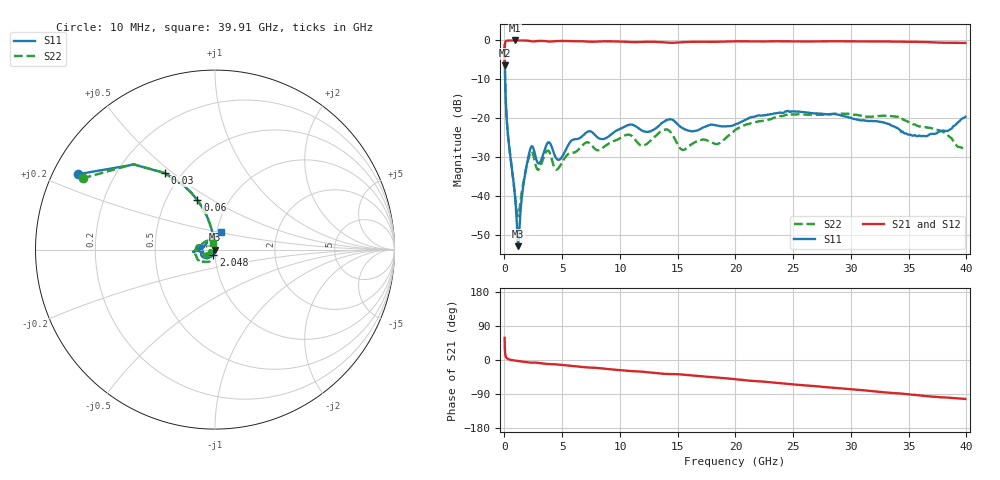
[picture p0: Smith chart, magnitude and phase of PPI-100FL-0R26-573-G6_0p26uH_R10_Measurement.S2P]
! Data measured by Modelithics Inc.  support@modelithics.com  813-866-6335  Tampa FL USA June 2025
! PPI-100FL-0R26-573-G6_0p26uH measured on 10-mil thick RO4350B board, mounted in 2-port shunt configuration on a 50-ohm transmission line
# Hz S MA R 50
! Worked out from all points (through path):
!   429 points, 10 MHz to 39.91 GHz, reference 50 ohm
!   highest |S21| = -0.03 dB at 882.5 MHz (marker M1); lowest = -6.4 dB at 10 MHz (marker M2)
!   group delay of S21, straight-line fit = 7.42 ps
!   lowest |S11| = -53.0 dB at 1.174 GHz (marker M3), VSWR 1.00, Z = 49.8 + j0.049 ohm
!   |S11| at or under -10 dB: 55.02 MHz to end of sweep
!   |S22| runs from -45.3 to -1.5 dB; largest |S21 - S12| = 0.024
!   S11 on the Smith chart (normalised r, x): 10 MHz: 0.07, +0.26; 30 MHz: 0.41, +0.47; 60 MHz: 0.71, +0.43; 2.048 GHz: 0.98, -0.06; 39.91 GHz: 1.05, +0.21
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1e7  0.8714 151.2  0.4784 58.5  0.4784 58.5  0.8372 151.7
3e7  0.5098 123.3  0.836 30.6  0.8361 30.6  0.5119 123.4
6e7  0.2921 109.5  0.9426 16.8  0.9427 16.8  0.2927 109.7
2e8  0.09232 98.5  0.9899 4.8  0.9899 4.8  0.09258 98.7
8.825328e8  0.01074 104.1  0.9961 -1.5  0.9962 -1.4  0.01119 113.4
1.173799e9  0.002238 167.3  0.9961 -2.7  0.9963 -2.7  0.005436 173.8
2.047598e9  0.0307 -106.3  0.9881 -6.3  0.9883 -6.3  0.0287 -132.0
2.435953e9  0.04288 -139.2  0.9679 -7.0  0.9681 -7.0  0.03559 -162.9
2.921397e9  0.02605 -141.1  0.9812 -7.7  0.9814 -7.7  0.02148 -155.4
3.795197e9  0.04875 -136.9  0.966 -10.6  0.966 -10.6  0.03811 -159.4
4.571907e9  0.02922 -143.5  0.9789 -11.8  0.9791 -11.8  0.02177 -149.8
6.70786e9  0.05777 -128.0  0.9723 -18.3  0.9724 -18.3  0.04383 -135.5
1.06885e10  0.08095 -150.5  0.9544 -28.9  0.9544 -28.9  0.06116 -145.7
1.204774e10  0.06749 -170.9  0.9557 -31.3  0.9558 -31.3  0.04421 -144.9
1.340699e10  0.08008 -169.7  0.9511 -35.5  0.9512 -35.6  0.0649 -139.3
1.41837e10  0.09562 177.0  0.933 -37.1  0.9332 -37.2  0.07013 -156.3
1.544585e10  0.07379 163.9  0.9477 -38.7  0.9477 -38.6  0.03886 -149.8
2.000902e10  0.08293 177.9  0.9717 -50.8  0.9718 -50.9  0.07064 -113.8
2.670815e10  0.115 -175.7  0.9678 -68.4  0.9678 -68.4  0.1097 -158.1
3.331019e10  0.0835 176.3  0.964 -86.2  0.9641 -86.3  0.107 175.0
3.641703e10  0.05848 128.1  0.9508 -94.9  0.9508 -94.7  0.07641 153.2
3.991223e10  0.1035 71.7  0.9264 -102.8  0.9265 -102.2  0.03802 111.0
